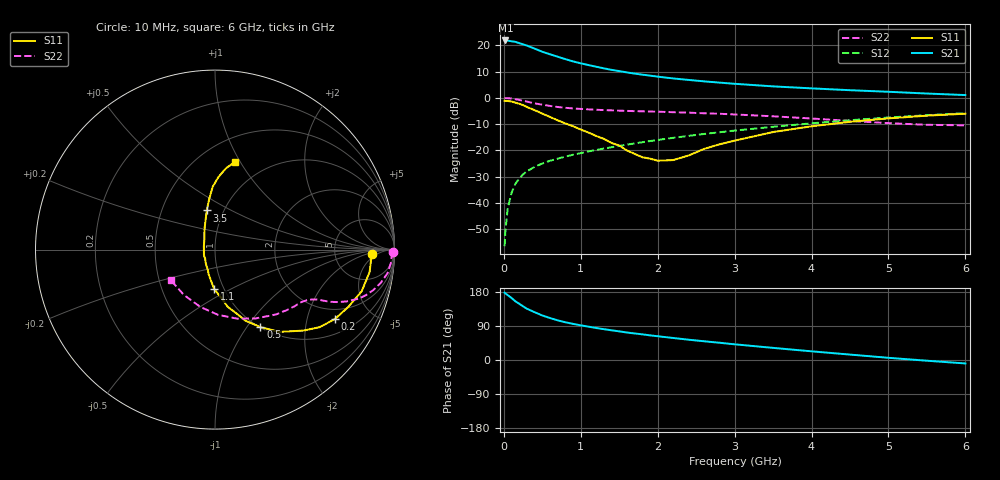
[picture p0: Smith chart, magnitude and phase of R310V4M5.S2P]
! SIEMENS Small Signal Semiconductors
! BFR181
! Si NPN RF Bipolar Junction Transistor in SOT23
! VCE = 10 V  IC = 4.5 mA
! Common Emitter S-Parameters:  May  1996
# GHz  S  MA  R  50
!  f  S11  S21  S12  S22
! GHz  MAG  ANG  MAG  ANG  MAG  ANG  MAG  ANG
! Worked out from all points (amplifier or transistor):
!   36 points, 10 MHz to 6 GHz, reference 50 ohm
!   highest |S21| = 21.8 dB at 20 MHz (marker M1)
!   |S21| within 3 dB of that: start of sweep to 391.2 MHz
!   unconditionally stable (mu >= 1): 1.269 GHz to 3.191 GHz
!   at 250 MHz: K = 0.37, MSG = 24.7 dB, |S12| = -29.1 dB
!   at 1.4 GHz: K = 1.02, MAG = 13.8 dB, |S12| = -18.8 dB
!   at 6 GHz: K = 0.87, MSG = 3.4 dB, |S12| = -5.8 dB
!   S11 on the Smith chart (normalised r, x): 10 MHz: 15, -3; 200 MHz: 1.55, -2.97; 500 MHz: 1.01, -1.16; 1.1 GHz: 0.90, -0.41; 3.5 GHz: 0.83, +0.38; 6 GHz: 0.73, +0.94
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0.01  0.8775 -1.6  12.32 177.5  0.0015 83.9  0.991 -0.8
0.02  0.8717 -3.2  12.35 175.7  0.0029 86.5  0.9853 -1.6
0.05  0.8706 -8.2  12.26 171.3  0.0078 85.5  0.9843 -4.0
0.1  0.8494 -15.9  11.91 163.7  0.0155 80.9  0.9701 -7.8
0.15  0.8083 -23.3  11.62 154.9  0.023 77.0  0.9416 -11.4
0.2  0.7714 -30.2  10.99 148.4  0.029 73.6  0.9109 -14.3
0.25  0.7251 -36.6  10.43 141.6  0.035 71.1  0.88 -16.7
0.3  0.669 -42.4  9.859 135.3  0.0399 68.8  0.8469 -18.8
0.4  0.5818 -52.0  8.646 126.1  0.0485 65.9  0.7854 -21.6
0.5  0.5006 -59.6  7.528 117.5  0.0562 63.9  0.7392 -23.3
0.6  0.4317 -66.7  6.739 110.7  0.0633 63.0  0.7006 -24.5
0.7  0.3731 -71.6  6.059 104.7  0.0695 62.7  0.6689 -25.2
0.8  0.3255 -77.6  5.441 99.6  0.0761 62.5  0.6452 -25.7
0.9  0.288 -80.7  4.932 95.3  0.0826 62.3  0.6286 -26.2
1.1  0.2182 -91.5  4.202 88.0  0.0954 62.7  0.6027 -27.5
1.3  0.1653 -99.1  3.636 81.4  0.1083 62.7  0.5845 -28.8
1.6  0.0994 -119.2  3.043 72.5  0.1287 62.7  0.5637 -31.2
2.2  0.0653 161.8  2.339 58.1  0.173 61.3  0.5324 -37.8
3.5  0.2231 101.9  1.651 32.0  0.281 53.0  0.4448 -59.6
4.5  0.3492 92.2  1.396 14.3  0.3742 43.3  0.3636 -87.4
5.5  0.4575 82.3  1.206 -1.9  0.4669 31.3  0.3064 -124.5
6  0.4986 77.4  1.128 -9.1  0.5103 24.6  0.2994 -145.5
